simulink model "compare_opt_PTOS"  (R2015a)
settings: Solver=ode5  StartTime=0.0  StopTime=trun  FixedStep=step_sz  RelTol=1e-3
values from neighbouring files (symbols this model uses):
  alpha = .5    (= 0.5)    [figure_4.m]    (also in figure_3.m = 0.8; figure_2.m; results.m = 0.7)
  bobar = 1.01*bo    (= 18458760)    [results.m]
  c = bo/w^2    (= 4.59233914625)    [figure_4.m]    (also in figure_3.m; figure_2.m; results.m)
  k1 = (c-xl)/(c*xl)    (= 1.95978557188)    [figure_4.m]    (also in figure_3.m = 0.508092555672; figure_2.m; results.m = 0.819169630574; switching_curves_comp_func.m = (c-xl)/(c*xl))
  k2 = sqrt(2*c*alpha*xl-alpha*xl^2)/(alpha*w*c*xl)    [figure_4.m]    (also in figure_3.m; figure_2.m; results.m; switching_curves_comp_func.m)
  step_sz = .00000006    (= 6e-08)    [figure_4.m]    (also in figure_2.m = 6e-07; results.m = 1e-07)
  T = 1    [figure_4.m]    (also in figure_3.m; figure_2.m; results.m; switching_curves_comp_func.m)
  w = 2*pi*3.175*10^2    (= 1994.91133503)    [figure_4.m]    (also in figure_3.m; figure_2.m; results.m; plotshaded.m = varargout)
  wbar = 0.99*w    (= 1974.96222168)    [results.m]
  x1Tol = .001*c    (= 0.00459233914625)    [figure_4.m]    (also in figure_2.m = 2.6e-12; results.m)
  x2Tol = .00001    (= 1e-05)    [figure_2.m]    (also in results.m = 9.16130941716)
  xl = .1*c    (= 0.459233914625)    [figure_4.m]    (also in figure_3.m = 1.37770174388; figure_2.m; results.m = 0.964391220713)
  Xo = [8.665 4229]    [figure_4.m]    (also in figure_3.m = [2*c, 0]; figure_2.m = [curves_optx1(k), curves_optx2(k)]; results.m = [3.0*c,0])
libraries: simulink x2, commnoisgen2 x1

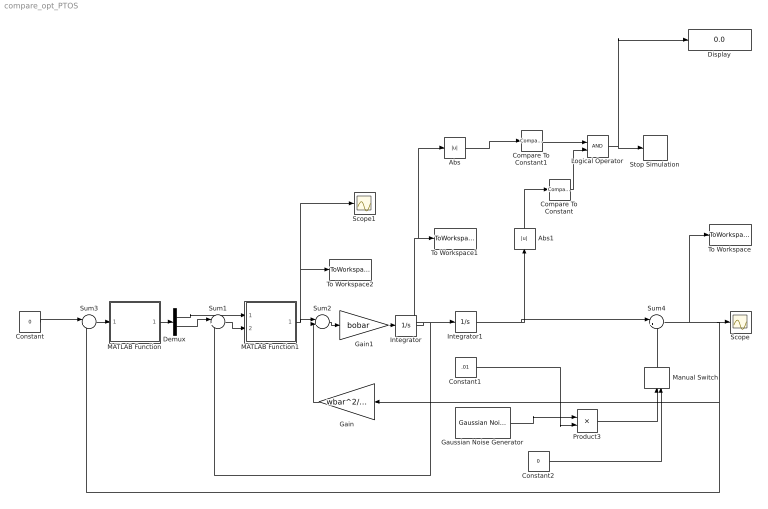
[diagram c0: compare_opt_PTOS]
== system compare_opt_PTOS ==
  Abs : Abs
  Abs1 : Abs
  Compare To Constant : simulink/Logic and Bit Operations/Compare To Constant  relop=<  const=x1Tol  OutDataTypeStr=boolean
  Compare To Constant1 : simulink/Logic and Bit Operations/Compare To Constant  relop=<  const=x2Tol  OutDataTypeStr=boolean
  Constant : Constant  Value=0
  Constant1 : Constant  Value=.01
  Constant2 : Constant  Value=0
  Demux : Demux  Outputs=2
  Display : Display
  Gain : Gain  Gain=wbar^2/bobar
  Gain1 : Gain  Gain=bobar
  Gaussian Noise Generator : commnoisgen2/Gaussian Noise Generator  m=0  d=1  s=41  Ts=step_sz  frameBased=off  sampPerFrame=1  orient=off  outDataType=double
  Integrator : Integrator  InitialCondition=Xo(2)
  Integrator1 : Integrator  InitialCondition=Xo(1)
  Logical Operator : Logic  AllPortsSameDT=off  OutDataTypeStr=boolean
  MATLAB Function : MATLAB Function  TreatAsAtomicUnit=on
  MATLAB Function1 : MATLAB Function  TreatAsAtomicUnit=on
  Manual Switch : ManualSwitch  CurrentSetting=0
  Product3 : Product
  Scope : Scope
  Scope1 : Scope
  Stop Simulation : Stop
  Sum1 : Sum  Inputs=|+-
  Sum2 : Sum  Inputs=|+-
  Sum3 : Sum  Inputs=|+-
  Sum4 : Sum  Inputs=|++
  To Workspace : ToWorkspace  VariableName=x1ptos  SampleTime=-1
  To Workspace1 : ToWorkspace  VariableName=x2ptos  SampleTime=-1
  To Workspace2 : ToWorkspace  VariableName=u_ptos  SampleTime=-1
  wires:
  Gain/1 -> Sum2/2
  Gain1/1 -> Integrator/1
  Sum2/1 -> Gain1/1
  Sum3/1 -> MATLAB Function/1(u)
  Constant/1 -> Sum3/1
  Integrator1/1 -> Abs1/1, Sum4/1
  Sum4/1 -> To Workspace/1, Gain/1, Sum3/2, Scope/1
  Constant1/1 -> Product3/2
  Manual Switch/1 -> Sum4/2
  Product3/1 -> Manual Switch/1
  Constant2/1 -> Manual Switch/2
  Integrator/1 -> Abs/1, To Workspace1/1, Sum1/2, Integrator1/1
  Compare To Constant1/1 -> Logical Operator/1
  Compare To Constant/1 -> Logical Operator/2
  Logical Operator/1 -> Display/1, Stop Simulation/1
  Abs/1 -> Compare To Constant1/1
  Abs1/1 -> Compare To Constant/1
  Sum1/1 -> MATLAB Function1/2(u)
  MATLAB Function/1(y) -> Demux/1
  Demux/2 -> Sum1/1
  Demux/1 -> MATLAB Function1/1(swtch)
  MATLAB Function1/1(y) -> Scope1/1, To Workspace2/1, Sum2/1
  Gaussian Noise Generator/1 -> Product3/1

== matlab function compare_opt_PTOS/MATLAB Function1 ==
function y = fcn(swtch, u, k2, T)
%#codegen

if(swtch ==0)
    control=sign(u);
else
    control=sat(u*k2, T);
end


y = [control];

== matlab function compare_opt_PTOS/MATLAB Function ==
function y = fcn(u, c, w, alpha, xl, k1, k2)
%#codegen
x1=-u;
if (mod(sign(u(1)/c)*floor(abs(u(1)/c)), 2)==0);
       x1_bar=c-abs(fracpart(u(1)/c)*c);
    else
        x1_bar=fracpart(u(1)/c)*c;
end

if( abs(u(1)) < 2*c & abs(u(1)) > xl )
      fx= sign(u(1)) *( w*sqrt(alpha*2*c*abs(u(1)) -alpha*u(1)^2) -1/k2);
      %control=sat( k2*(-Fptos -u(2)), T);
      swtch=1;
 elseif(abs(u(1)) <xl )
     fx=(k1/k2)*u(1);
    % control=sat( k2*(-Fptos -u(2)), T);
    swtch=1;
else
     fx=sign(u(1))*w*sqrt(c^2 -x1_bar^2 );
     swtch=0;
end





y = [swtch fx];
